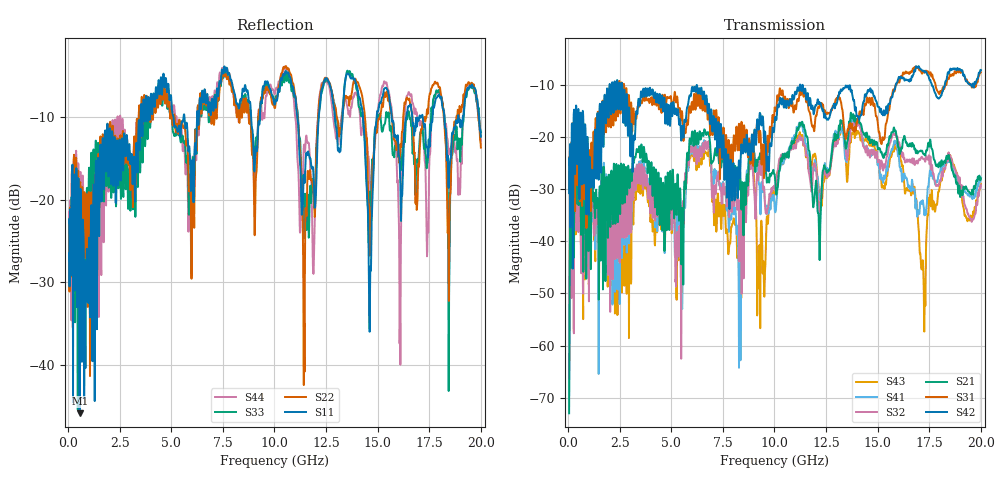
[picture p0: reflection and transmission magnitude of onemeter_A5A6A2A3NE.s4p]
! FILE: D:\iPass\iPassCable1005\iPassCable\SOLT_cal\onemeter_A5A6A2A3NE.s4p
# MHz S MA R 50.00
! FREQ  S11  S12  S13  S14
!  S21  S22  S23  S24
!  S31  S32  S33  S34
!  S41  S42  S43  S44
!  MAG  ANG  MAG  ANG  MAG  ANG  MAG  ANG
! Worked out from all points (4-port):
!   1996 points, 50 MHz to 20 GHz, reference 50 ohm
!   strongest paths, dB at 50 MHz, 5.04 GHz, 10.03 GHz, 15.02 GHz, 20 GHz:
!     S42: -24.1, -16.0, -16.2, -14.2, -7.1
!     S31: -23.9, -13.8, -14.4, -17.9, -7.5
!     S21: -73.0, -29.4, -28.0, -22.3, -27.9
!     S32: -66.2, -36.8, -30.0, -24.6, -29.2
!     S41: -69.5, -32.7, -34.4, -25.1, -27.7
!     S43: -63.8, -36.3, -29.8, -24.5, -29.0
!   lowest |S11| = -45.8 dB at 560 MHz (marker M1), VSWR 1.01, Z = 50.5 + j0.00411 ohm
!   |S11| at or under -10 dB: start of sweep to 3.515 GHz; 11.11 GHz to 12.15 GHz (1.039 GHz wide, 8.94 % of centre); 15.68 GHz to 16.38 GHz (705.8 MHz wide, 4.4 % of centre)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
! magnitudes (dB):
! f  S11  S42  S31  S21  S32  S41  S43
! 50 MHz  -22.4  -24.1  -23.9  -73.0  -66.2  -69.5  -63.8
! 560 MHz  -45.8  -24.8  -27.6  -26.8  -32.4  -28.6  -33.2
! 6.66 GHz  -8.0  -13.5  -14.5  -18.9  -20.8  -21.0  -22.8
! 8.31 GHz  -8.6  -27.1  -19.3  -27.6  -38.3  -42.9  -45.7
! 13.9 GHz  -5.5  -14.9  -18.0  -16.1  -17.5  -17.8  -20.0
! 17.23 GHz  -10.9  -7.2  -7.4  -23.3  -24.2  -33.3  -48.7
! 20 GHz  -12.4  -7.1  -7.5  -27.9  -29.2  -27.7  -29.0
